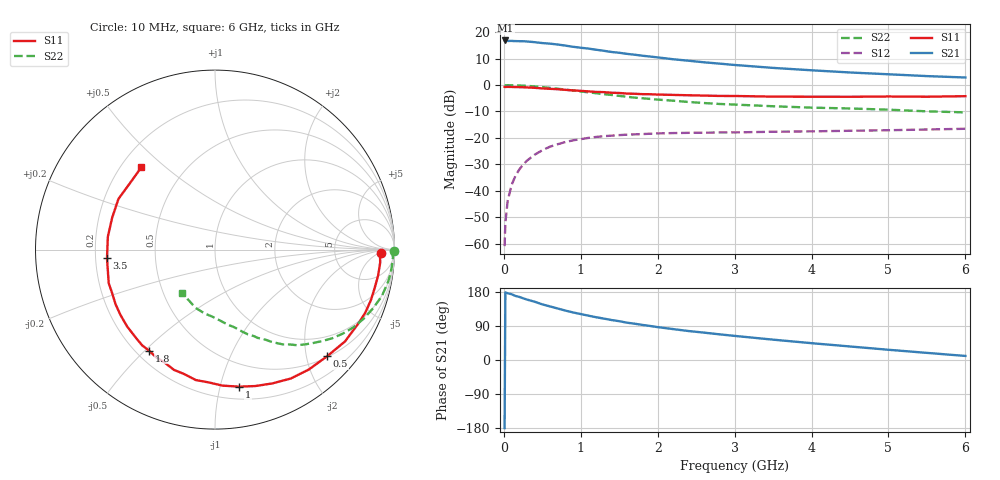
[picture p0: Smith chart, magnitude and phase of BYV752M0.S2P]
! SIEMENS Small Signal Semiconductors
! BFY420
! Si NPN RF SIEGET Grounded Emitter Transistor in MICRO-X
! VCE = 0.75 V  IC = 2 mA
! Common Emitter S-Parameters:  October  1996
# GHz  S  MA  R  50
!  f  S11  S21  S12  S22
! GHz  MAG  ANG  MAG  ANG  MAG  ANG  MAG  ANG
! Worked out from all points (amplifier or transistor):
!   36 points, 10 MHz to 6 GHz, reference 50 ohm
!   highest |S21| = 16.9 dB at 20 MHz (marker M1)
!   |S21| within 3 dB of that: start of sweep to 1.078 GHz
!   unconditionally stable (mu >= 1): 3.928 GHz to end of sweep
!   at 250 MHz: K = 0.05, MSG = 23.3 dB, |S12| = -30.1 dB
!   at 1.4 GHz: K = 0.33, MSG = 15.8 dB, |S12| = -19.1 dB
!   at 6 GHz: K = 1.28, MAG = 6.5 dB, |S12| = -16.5 dB
!   S11 on the Smith chart (normalised r, x): 10 MHz: 24, -6; 500 MHz: 0.52, -2.41; 1 GHz: 0.30, -1.15; 1.8 GHz: 0.25, -0.52; 3.5 GHz: 0.25, -0.04; 6 GHz: 0.28, +0.42
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0.01  0.9239 -1.2  6.951 -179.6  0.0009 105.7  0.9952 -0.5
0.02  0.9199 -2.0  6.959 178.4  0.0025 98.8  0.987 -1.0
0.05  0.9232 -4.5  6.808 176.1  0.0065 84.8  0.9926 -2.5
0.1  0.9203 -9.0  6.818 173.6  0.0128 85.0  0.9896 -5.3
0.15  0.9149 -13.6  6.768 169.1  0.0191 81.3  0.987 -7.9
0.25  0.9081 -22.7  6.734 162.9  0.0313 76.2  0.9722 -13.0
0.3  0.8994 -26.9  6.656 159.5  0.0372 74.5  0.9653 -15.5
0.4  0.8869 -35.2  6.459 153.8  0.0481 69.0  0.9401 -20.3
0.5  0.8624 -43.5  6.21 146.8  0.0586 64.4  0.9134 -24.9
0.7  0.8333 -59.5  5.831 135.9  0.0761 55.4  0.8523 -33.3
0.8  0.8109 -66.9  5.56 130.4  0.0836 51.1  0.819 -37.1
1  0.7753 -80.0  5.069 121.2  0.0949 44.2  0.7557 -43.5
1.1  0.7591 -86.8  4.887 117.0  0.1002 41.2  0.7274 -46.6
1.4  0.7146 -103.8  4.214 105.5  0.1104 33.0  0.6496 -54.4
1.6  0.6886 -114.2  3.885 98.5  0.1153 28.9  0.6003 -58.7
1.8  0.6724 -123.1  3.582 92.6  0.1184 25.5  0.5631 -62.0
2.2  0.6507 -138.7  3.073 81.6  0.1235 19.6  0.5056 -68.9
2.8  0.6222 -157.2  2.543 67.8  0.127 14.1  0.4391 -77.2
3.5  0.6037 -175.4  2.108 53.7  0.131 10.0  0.3971 -85.7
4.5  0.5999 162.7  1.727 35.7  0.1366 5.2  0.3604 -99.3
5.5  0.6015 141.5  1.475 18.8  0.1444 2.3  0.3183 -117.3
6  0.6154 131.8  1.388 10.7  0.149 1.0  0.3042 -127.8
